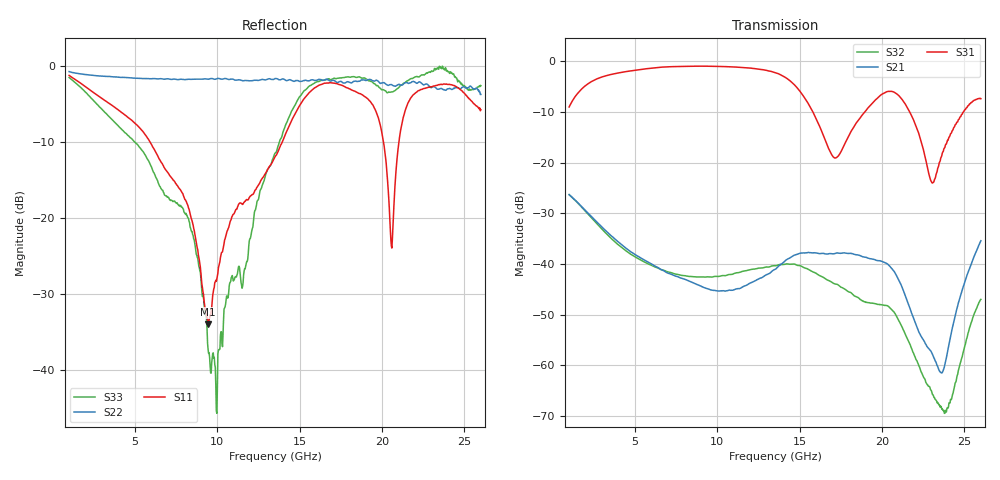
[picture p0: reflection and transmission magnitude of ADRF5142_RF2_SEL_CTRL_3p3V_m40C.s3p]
! Device: ADRF5142
! Description: Silicon, SPDT Switch, Reflective
! Frequency: 8.00 GHz - 11.00 GHz
! Ports:
!  RFC = Port 1
!  RF1 = Port 2
!  RF2 = Port 3
! VDD = +3.3V
! VSS = -3.3V
! CTRL = +3.3V
! Temp = -40C
! Data:  Data was collected using an calibrated 4 port network analyzer.
!  The reference plane is the package pins of ADRF5142 switch.
! Notes: Analog Devices supplies this data as a sample of measured data
!  for this product.  Your particular data for this product may vary.
!  Data was taken at -40 degrees C.
!  Analog Devices reserves the right to change this data at anytime.
# HZ S DB R 50
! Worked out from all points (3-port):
!   801 points, 1 GHz to 26 GHz, reference 50 ohm
!   strongest paths, dB at 1 GHz, 7.25 GHz, 13.5 GHz, 19.75 GHz, 26 GHz:
!     S31: -9.0, -1.0, -2.2, -7.2, -7.4
!     S21: -26.3, -42.1, -41.0, -39.3, -35.4
!     S32: -26.3, -41.7, -40.3, -48.0, -47.0
!   lowest |S11| = -34.0 dB at 9.438 GHz (marker M1), VSWR 1.04, Z = 50.7 - j1.87 ohm
!   |S11| at or under -10 dB: 5.919 GHz to 13.94 GHz (8.018 GHz wide, 80.8 % of centre); 20.09 GHz to 21.02 GHz (930.5 MHz wide, 4.53 % of centre)
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1e9  -1.20 158.5  -26.30 -41.6  -9.00 38.4
     -26.30 -41.6  -0.69 170.0  -26.31 -60.6
     -9.00 38.4  -26.31 -60.6  -1.47 122.5
2.8437e9  -4.02 131.6  -32.21 -87.8  -3.25 -17.3
          -32.21 -87.8  -1.27 154.9  -32.56 -142.6
          -3.25 -17.3  -32.56 -142.6  -5.35 31.8
5.875e9  -9.83 95.2  -39.73 -116.5  -1.38 -90.7
         -39.73 -116.5  -1.63 133.8  -40.08 137.0
         -1.38 -90.7  -40.08 137.0  -12.70 -82.6
9.4375e9  -34.01 -67.7  -44.91 -133.2  -0.96 -173.8
          -44.91 -133.2  -1.71 104.7  -42.51 61.7
          -0.96 -173.8  -42.51 61.7  -37.32 -114.8
1.35e10  -11.93 -109.7  -41.04 -144.5  -2.20 80.3
         -41.04 -144.5  -1.61 74.1  -40.31 -38.1
         -2.20 80.3  -40.31 -38.1  -11.46 42.1
1.71562e10  -2.23 166.8  -37.90 136.2  -19.06 36.0
            -37.90 136.2  -1.96 48.8  -43.94 -164.1
            -19.06 36.0  -43.94 -164.1  -1.60 -98.3
2.05625e10  -23.65 -28.5  -40.77 49.0  -5.92 -9.9
            -40.77 49.0  -2.39 19.7  -48.94 64.3
            -5.92 -9.9  -48.94 64.3  -3.38 -164.2
2.2e10  -3.56 168.2  -51.47 28.1  -12.26 -71.4
        -51.47 28.1  -2.09 6.5  -58.28 -5.6
        -12.26 -71.4  -58.28 -5.6  -1.39 179.9
2.35937e10  -2.35 91.4  -61.47 114.5  -18.87 -0.2
            -61.47 114.5  -2.90 -8.6  -68.17 -67.1
            -18.87 -0.2  -68.17 -67.1  -0.28 143.6
2.6e10  -5.72 -2.4  -35.40 161.6  -7.36 -51.8
        -35.40 161.6  -3.70 -22.2  -46.97 134.2
        -7.36 -51.8  -46.97 134.2  -2.54 83.1
